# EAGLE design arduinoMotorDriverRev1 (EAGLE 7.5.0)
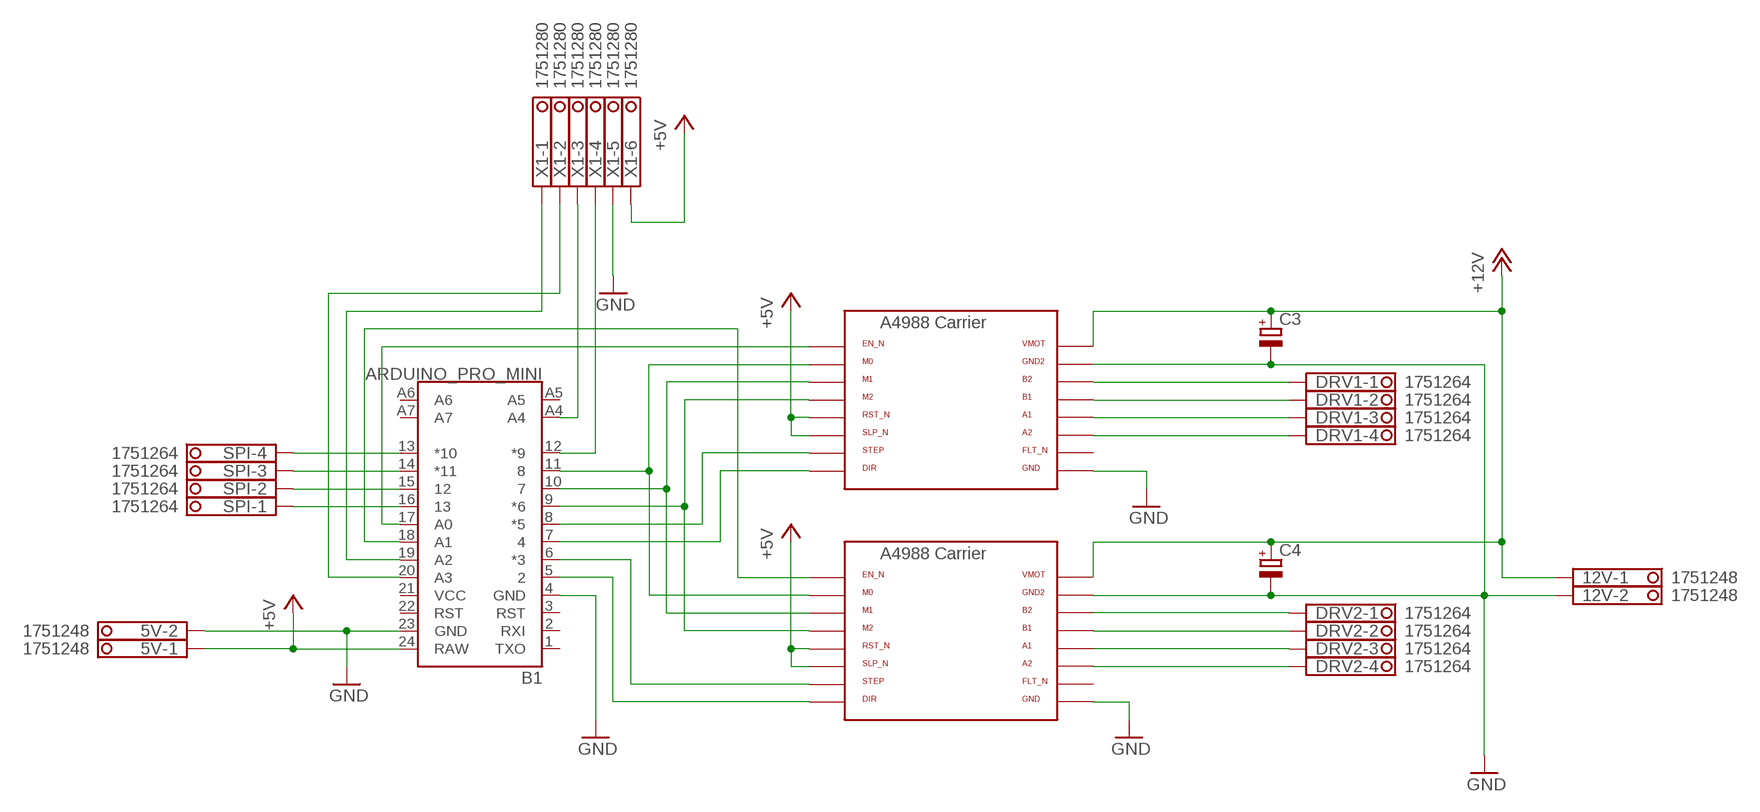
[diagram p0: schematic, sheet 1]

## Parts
5V  1751248  [1751248]
12V  1751248  [1751248]
B1  ARDUINO_PRO_MINI  [ARDUINO_PRO_MINI]
C3  CPOL-EUE3.5-10  [E3,5-10]
C4  CPOL-EUE3.5-10  [E3,5-10]
DRV1  1751264  [1751264]
DRV2  1751264  [1751264]
SPI  1751264  [1751264]
U$4  A4988BREAKOUT  [A4988BREAKOUT]
U$5  POLOLU_A4983CARRIER  [A4988BREAKOUT]
X1  1751280  [1751280]

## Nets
+5V: 5V.1 B1.24(RAW) U$4.RST(RST_N) U$4.SLP(SLP_N) U$5.RST(RST_N) U$5.SLP(SLP_N) X1.6
+12V: 12V.1 C3.+ C4.+ U$4.VMOT U$5.VMOT
GND: 5V.2 12V.2 B1.4(GND) B1.23(GND) C3.- C4.- U$4.GND(GND2) U$4.GND@0(GND) U$5.GND(GND2) U$5.GND@0(GND) X1.5
N$1: B1.11 U$4.MS1(M0) U$5.MS1(M0)
N$2: B1.17(A0) U$4.EN(EN_N)
N$3: B1.9(*6) U$4.MS3(M2) U$5.MS3(M2)
N$4: B1.13(*10) SPI.4
N$5: B1.8(*5) U$4.STEP
N$6: B1.7 U$4.DIR
N$7: B1.10 U$4.MS2(M1) U$5.MS2(M1)
N$8: B1.14(*11) SPI.3
N$9: B1.6(*3) U$5.STEP
N$10: B1.5 U$5.DIR
N$11: DRV1.4 U$4.1B(A2)
N$12: DRV1.3 U$4.1A(A1)
N$13: DRV1.2 U$4.2A(B1)
N$14: DRV1.1 U$4.2B(B2)
N$15: DRV2.4 U$5.1B(A2)
N$16: DRV2.3 U$5.1A(A1)
N$17: DRV2.2 U$5.2A(B1)
N$18: DRV2.1 U$5.2B(B2)
N$19: B1.15 SPI.2
N$20: B1.18(A1) U$5.EN(EN_N)
N$21: B1.12(*9) X1.4
N$22: B1.16 SPI.1
N$23: B1.19(A2) X1.1
N$24: B1.20(A3) X1.2
N$25: B1.A4 X1.3
Unconnected: B1.1(TXO) B1.2(RXI) B1.3(RST) B1.22(RST) B1.A5 B1.A6 B1.A7 U$4.VDD(FLT_N) U$5.VDD(FLT_N)

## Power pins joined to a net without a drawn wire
VCC: B1.21(VCC)

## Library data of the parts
5V 12V = con-phoenix-350:1751248: MKDS 1/ 2-3,5 Printklemme; OC_FARNELL: unknown; OC_NEWARK: unknown
B1 = SparkFun-Boards:ARDUINO_PRO_MINI: SparkFun Pro Mini Pro Mini compatible footprint. Dimensions: 0.7 x 1.3" PCB Thickness: 0.8mm SparkFun Products: 3.3V/8MHz 5V/16MHz
C3 C4 = rcl:CPOL-EU: POLARIZED CAPACITOR, European symbol
DRV1 DRV2 SPI = con-phoenix-350:1751264: MKDS 1/ 4-3,5 Printklemme Nennstrom: 10 A Bemessungsspannung: 160 V Raster: 3,5 mm Polzahl: 4 Montageart: Löten Anschlussart: Schraubanschluss Anschlussrichtung vom Leiter zur Platine: 0° Source: http://eshop.phoenixcontact.com .. 1751264.pdf; MPN: 1751264; OC_FARNELL: unknown; OC_NEWARK: 10R0934
U$4 = RepRapjr:A4988BREAKOUT
U$5 = RepRapjr:POLOLU_A4983CARRIER
X1 = con-phoenix-350:1751280: MKDS 1/ 6-3,5 Printklemme Nennstrom: 10 A Bemessungsspannung: 160 V Raster: 3,5 mm Polzahl: 6 Montageart: Löten Anschlussart: Schraubanschluss Anschlussrichtung vom Leiter zur Platine: 0° Source: http://eshop.phoenixcontact.com .. 1751280.pdf; MPN: 1751280; OC_FARNELL: unknown; OC_NEWARK: 27R1765

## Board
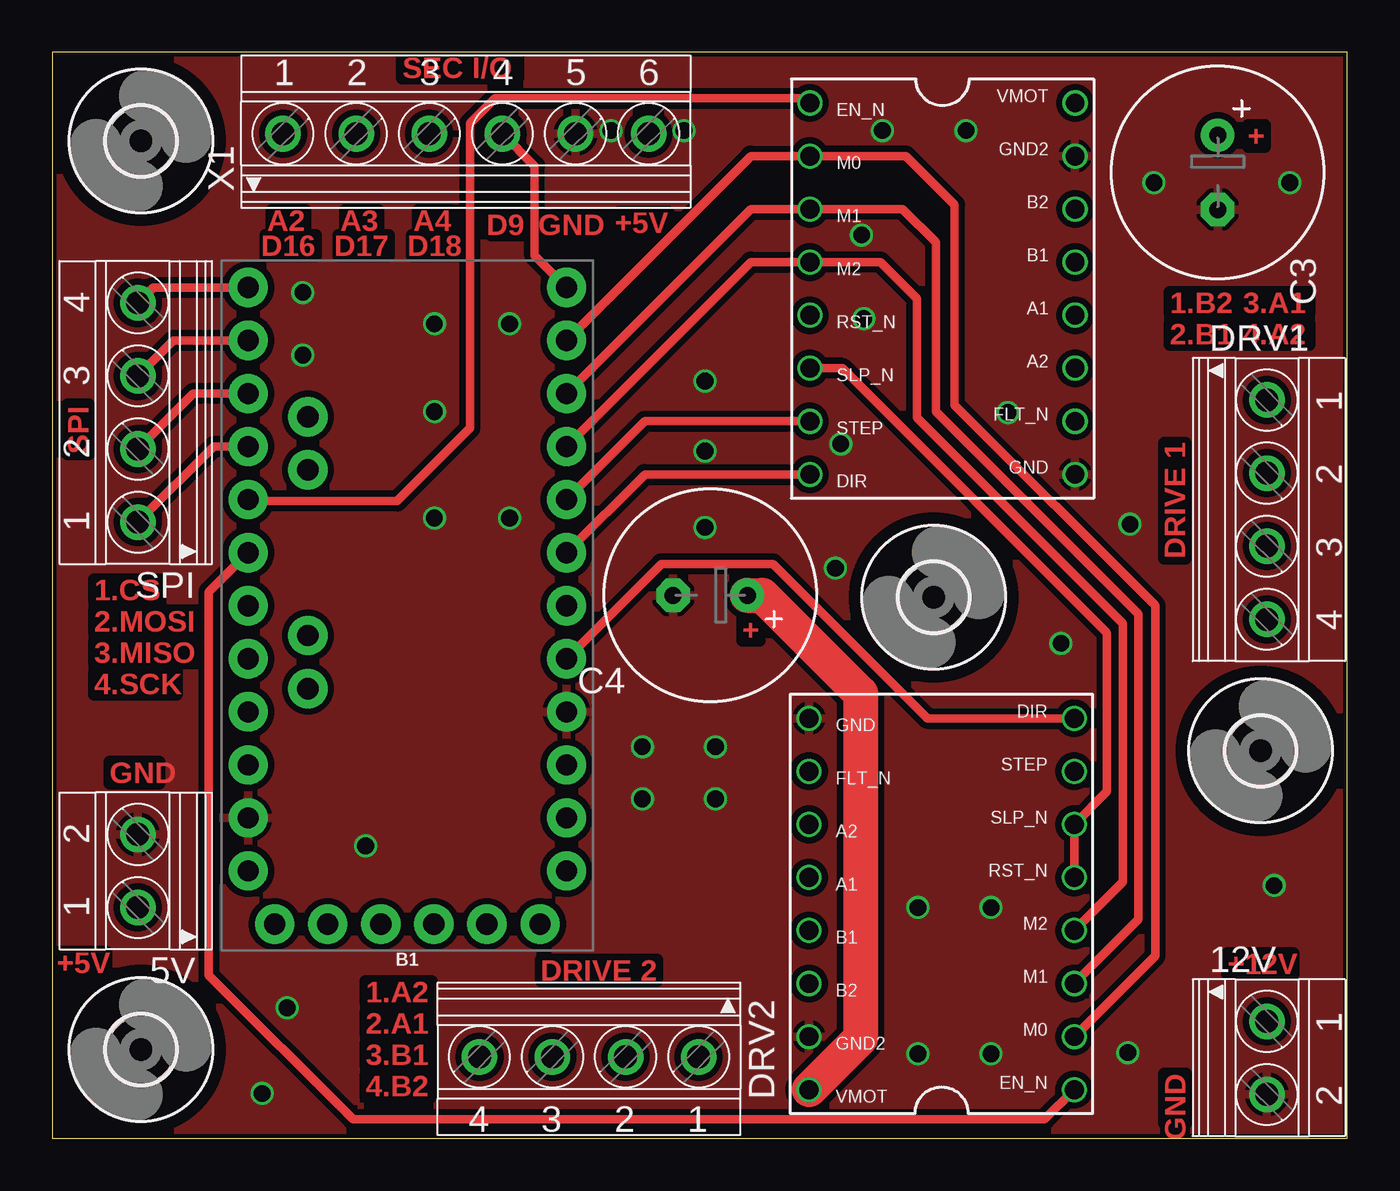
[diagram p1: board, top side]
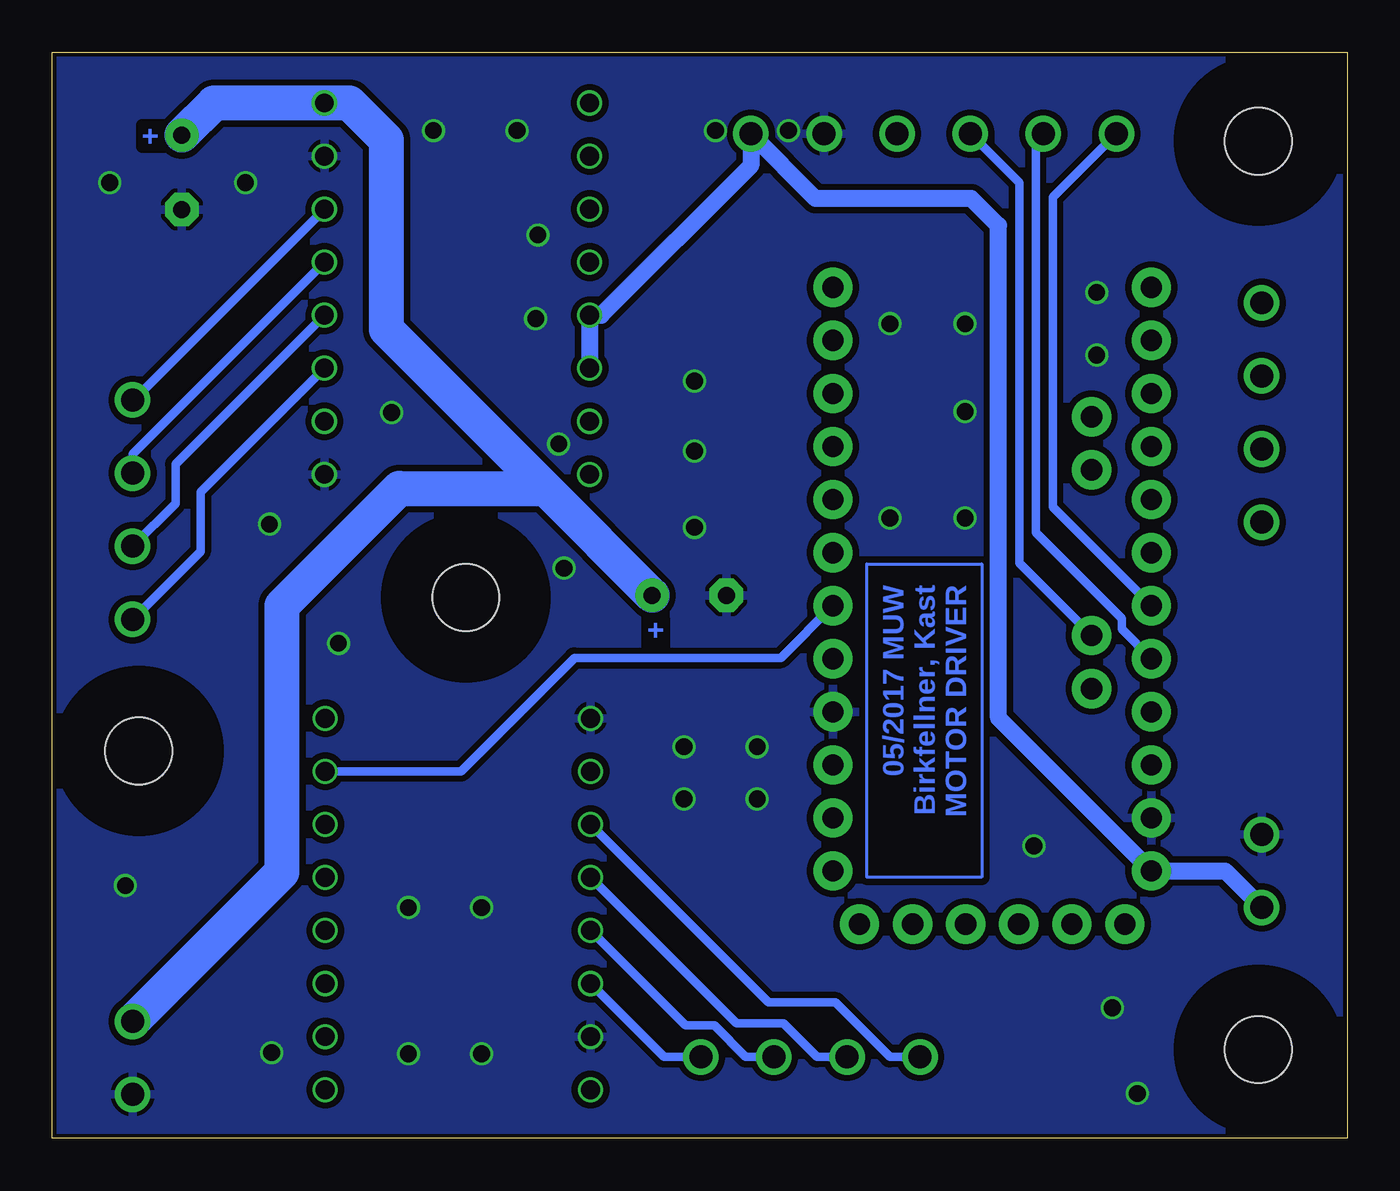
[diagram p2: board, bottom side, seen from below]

Size 62 x 52 mm. Coordinates in mm from the lower left corner, seen from the top.
Outline: 0,0 62,0 62,52 0,52 0,0
Copper layers (1*16): Top 0.035mm / dielectric 1.5mm / Bottom 0.035mm
Design rules "Eagle-DRU - 1506 - LeitOn - 01 and 02 layers - STANDARD *": minimum track width 0.15mm, minimum drill 0.3mm, track to track 0.3mm, track to pad 0.3mm, pad to pad 0.3mm, via to via 0.3mm, smd to smd 0.3mm, copper to edge 0.2mm, drill to drill 0.25mm, minimum pad ring 0.15mm, minimum via ring 0.15mm, stop-mask expansion 0.05mm, vias tented up to drill 0mil, thermal gap 0.2mm

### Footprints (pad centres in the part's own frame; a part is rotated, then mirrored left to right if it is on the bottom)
1751248 = drill 1.1 pad 1.7: 1 -1.75,-0.1; 2 1.75,-0.1
ARDUINO_PRO_MINI = drill 1.016 pad 1.88: 1 -7.62,12.7; 2 -7.62,10.16; 3 -7.62,7.62; 4 -7.62,5.08; 5 -7.62,2.54; 6 -7.62,0; 7 -7.62,-2.54; 8 -7.62,-5.08; 9 -7.62,-7.62; 10 -7.62,-10.16; 11 -7.62,-12.7; 12 -7.62,-15.24; 13 7.62,-15.24; 14 7.62,-12.7; 15 7.62,-10.16; 16 7.62,-7.62; 17 7.62,-5.08; 18 7.62,-2.54; 19 7.62,0; 20 7.62,2.54; 21 7.62,5.08; 22 7.62,7.62; 23 7.62,10.16; 24 7.62,12.7; A4 4.763,1.429; A5 4.763,3.969; A6 4.763,-9.049; A7 4.763,-6.509; BLK -6.35,15.24; GND -3.81,15.24; GRN 6.35,15.24; RXI 1.27,15.24; TXO 3.81,15.24; VCC -1.27,15.24
E3,5-10 = drill 0.813 pad 1.6: + -1.778,0 | drill 0.813 pad 1.6 octagon: - 1.778,0
1751264 = drill 1.1 pad 1.7: 1 -5.25,-0.1; 2 -1.75,-0.1; 3 1.75,-0.1; 4 5.25,-0.1
3,2 = hole 3.2: 0,0
A4988BREAKOUT = drill 0.9: 1A 8.89,1.27; 1B 11.43,1.27; 2A 6.35,1.27; 2B 3.81,1.27; DIR 16.51,-11.43; EN -1.27,-11.43; GND 16.51,1.27; GND@0 1.27,1.27; MS1 1.27,-11.43; MS2 3.81,-11.43; MS3 6.35,-11.43; RST 8.89,-11.43; SLP 11.43,-11.43; STEP 13.97,-11.43; VDD 13.97,1.27; VMOT -1.27,1.27
1751280 = drill 1.1 pad 1.7: 1 -8.75,-0.1; 2 -5.25,-0.1; 3 -1.75,-0.1; 4 1.75,-0.1; 5 5.25,-0.1; 6 8.75,-0.1

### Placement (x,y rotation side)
5V  4,12.8 90 top
12V  58.25,3.85 270 top
B1  17,25.5 180 top
C3  55.8,46.25 270 top
C4  31.5,26 180 top
DRV1  58.25,30.1 270 top
DRV2  25.7,3.8 180 top
SPI  4,34.75 90 top
U$1  [3,2]  42.2,25.9 0 top
U$2  [3,2]  4.25,47.75 0 top
U$3  [3,2]  57.85,18.55 0 top
U$4  47.7,48.3 270 top
U$5  37.5,3.6 90 top
U$6  [3,2]  4.25,4.25 0 top
X1  19.8,48.2 0 top

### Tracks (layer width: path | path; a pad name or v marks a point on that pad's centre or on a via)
+5V
  Top 0.406: U$4.SLP 37.83,36.87 50.5,24.2 50.5,16.6 U$5.SLP U$5.RST
  Bottom 0.813: 5V.1 5.85,12.8 B1.24 16.7,20.12 16.7,43.7 18,45 25.45,45 X1.6 28.55,46.58 35.72,39.41 U$4.RST U$4.SLP
+12V
  Top 1.676: C4.+ 34,26 38.7,21.3 38.7,4.8 U$5.VMOT
  Bottom 1.676: 12V.1 51,12.75 51,25.5 45.39,31.11 38.39,31.11 | 38.39,31.11 46,38.72 46,47.8 47.77,49.57 U$4.VMOT 54.26,49.57 C3.+ | 38.39,31.11 C4.+
GND  (via drill 0.8)
  other vias: 28.25,18.75 31.75,18.75 31.75,16.25 28.25,16.25 26.75,48.25 30.25,48.25 38.75,43.25 38.85,39.25 31.25,32.9 37.5,27.3 48.3,23.7 39.75,48.25 43.75,48.25 15,14 21.9,39 44.95,11.05 41.45,11.05 41.45,4.05 44.95,4.05 58.5,12.1 51.5,4.1 52.75,45.75 59.25,45.75 31.25,29.25 31.25,36.25 37.75,33.25 51.6,29.4 45.75,34.75 11.25,6.25 10.05,2.15 12,37.5 12,40.5 18.3,39 18.3,34.8 18.3,29.7 21.9,29.7
  pour Bottom: 0,52 62,52 62,0 0,0
  pour Top: 0,52 62,52 62,0 0,0
N$1
  Top 0.406: B1.11 33.45,47.03 U$4.MS1 40.87,47.03 43.2,44.7 43.2,35.1 52.8,25.5 52.8,8.74 U$5.MS1
N$2
  Top 0.406: B1.17 9.46,30.5 16.5,30.5 20,34 20,48.6 21.2,49.8 36.04,49.8 U$4.EN
N$3
  Top 0.406: B1.9 33.45,41.95 U$4.MS3 39.65,41.95 41.4,40.2 41.4,34.5 51.25,24.65 51.25,12.27 U$5.MS3
N$4
  Top 0.406: B1.13 4.84,40.74 SPI.4
N$5
  Top 0.406: B1.8 28.37,34.33 U$4.STEP
N$6
  Top 0.406: B1.7 28.37,31.79 U$4.DIR
N$7
  Top 0.406: B1.10 33.45,44.49 U$4.MS2 40.71,44.49 42.3,42.9 42.3,34.8 52,25.1 52,10.48 U$5.MS2
N$8
  Top 0.406: B1.14 5.8,38.2 SPI.3
N$9
  Bottom 0.406: B1.6 27.12,23 37,23 42.43,17.57 U$5.STEP
N$10
  Top 0.406: B1.5 29.16,27.5 34.5,27.5 41.89,20.11 U$5.DIR
N$11
  Bottom 0.406: U$4.1B 54.9,30.94 54.9,28.1 DRV1.4
N$12
  Bottom 0.406: U$4.1A 56.1,32.28 56.1,30.4 DRV1.3
N$13
  Bottom 0.406: U$4.2A 58.15,32.77 DRV1.2
N$14
  Bottom 0.406: U$4.2B 58.11,35.35 DRV1.1
N$15
  Bottom 0.406: DRV2.4 21.9,3.9 24.5,6.5 27.7,6.5 U$5.1B
N$16
  Bottom 0.406: DRV2.3 25.4,3.9 27,5.5 29.24,5.5 U$5.1A
N$17
  Bottom 0.406: DRV2.2 28.8,3.9 30.3,5.4 31.68,5.4 U$5.2A
N$18
  Bottom 0.406: U$5.2B 32.72,3.9 DRV2.1
N$19
  Top 0.406: B1.15 6.76,35.66 SPI.2
N$20
  Top 0.406: B1.18 7.5,26.16 7.5,7.8 14.4,0.9 47.5,0.9 U$5.EN
N$21
  Top 0.406: B1.12 23.1,42.26 23.1,46.55 X1.4
N$22
  Top 0.406: B1.16 7.72,33.12 SPI.1
N$23
  Bottom 0.406: B1.19 14.1,30.22 14.1,45.05 X1.1
N$24
  Bottom 0.406: B1.20 10.8,24.38 10.8,24.9 14.9,29 14.9,47.75 X1.2
N$25
  Bottom 0.406: B1.A4 15.7,27.53 15.7,45.75 X1.3
N$60
  Bottom 0.152: 17.5,27.5 17.5,12.5 23,12.5 23,27.5 17.5,27.5

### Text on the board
Top: SEC I/O | + | A2 | A3 | A4 | D9 | GND | +5V | D16 | D17 | D18 | 1.B2 | 3.A1 | 2.B1 | 4.A2 | SPI | DRIVE 1 | 1.CS | + | 2.MOSI | 3.MISO | 4.SCK | GND | DRIVE 2 | +5V | +12V | 1.A2 | 2.A1 | 3.B1 | GND | 4.B2
Bottom: + | MOTOR DRIVER | Birkfellner, Kast | 05/2017 MUW | +

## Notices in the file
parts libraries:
SparkFun-Boards: Licensing: Creative Commons ShareAlike 4.0 International - https://creativecommons.org/licenses/by-sa/4.0
